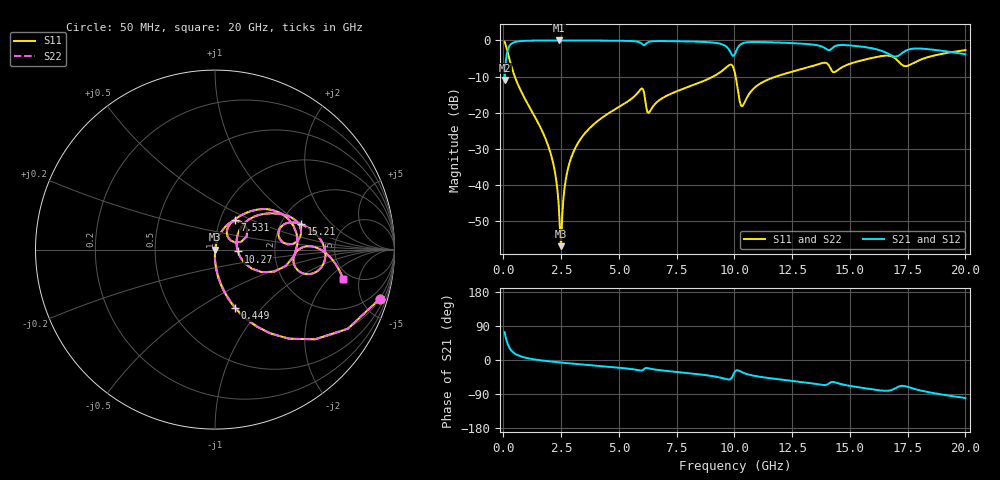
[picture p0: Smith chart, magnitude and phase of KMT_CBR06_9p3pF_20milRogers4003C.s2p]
! Data measured by Modelithics Inc. support@modelithics.com 813-866-6335
! KEMET CBR0603 9.3pF, Pad Width= 0.851mm, Pad Length= 0.64mm, Pad Gap= 0.62mm, 20mil Rogers 4003C substrate Data, January 2022
# hz S ma R 50
! 2 Port Network Data from SP1.SP block
! freq  magS11  angS11  magS21  angS21  magS12  angS12  magS22  angS22
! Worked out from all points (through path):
!   401 points, 50 MHz to 20 GHz, reference 50 ohm
!   highest |S21| = -0.01 dB at 2.394 GHz (marker M1); lowest = -11.0 dB at 50 MHz (marker M2)
!   group delay of S21, straight-line fit = 14.5 ps
!   lowest |S11| = -57.0 dB at 2.494 GHz (marker M3), VSWR 1.00, Z = 50.1 + j0.0514 ohm
!   |S11| at or under -10 dB: 489.8 MHz to 9.08 GHz (8.59 GHz wide, 180 % of centre); 10.05 GHz to 11.81 GHz (1.753 GHz wide, 16 % of centre)
!   |S22| runs from -57.0 to -0.4 dB; largest |S21 - S12| = 0
!   S11 on the Smith chart (normalised r, x): 50 MHz: 0.99, -6.73; 449 MHz: 0.99, -0.73; 7.531 GHz: 1.17, +0.41; 10.27 GHz: 1.29, -0.03; 15.21 GHz: 2.57, +0.97; 20 GHz: 4.24, -3.05
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5e7  0.9591 -16.6  0.2826 73.4  0.2826 73.4  0.9591 -16.6
2.495e8  0.5584 -56.7  0.8288 33.3  0.8288 33.3  0.5584 -56.7
4.49e8  0.3435 -71.0  0.9384 18.9  0.9384 18.9  0.3435 -71.0
1.94525e9  0.03417 -91.4  0.9982 -3.3  0.9982 -3.3  0.03417 -91.4
2.2445e9  0.01412 -90.4  0.9986 -5.3  0.9986 -5.3  0.01412 -90.4
2.394125e9  0.005202 -82.5  0.9987 -6.2  0.9987 -6.2  0.005202 -82.5
2.493875e9  0.001418 21.2  0.9987 -6.8  0.9987 -6.8  0.001418 21.2
2.843e9  0.01932 77.3  0.9984 -8.8  0.9984 -8.8  0.01932 77.3
3.391625e9  0.04567 76.4  0.9974 -11.8  0.9974 -11.8  0.04567 76.4
5.93525e9  0.2096 48.0  0.9271 -27.7  0.9271 -27.7  0.2096 48.0
6.284375e9  0.09914 40.8  0.9506 -22.0  0.9506 -22.0  0.09914 40.8
6.73325e9  0.1477 59.8  0.9796 -26.6  0.9796 -26.6  0.1477 59.8
7.53125e9  0.1993 56.8  0.9745 -31.7  0.9745 -31.7  0.1993 56.8
9.52625e9  0.3924 33.8  0.8682 -48.5  0.8682 -48.5  0.3924 33.8
1.0025e10  0.3518 -20.4  0.6513 -30.4  0.6513 -30.4  0.3518 -20.4
1.027438e10  0.1275 -4.8  0.8834 -30.7  0.8834 -30.7  0.1275 -4.8
1.336662e10  0.4412 25.5  0.877 -61.9  0.877 -61.9  0.4412 25.5
1.416462e10  0.4075 4.1  0.7473 -59.1  0.7473 -59.1  0.4075 4.1
1.5212e10  0.4987 16.5  0.84 -70.4  0.84 -70.4  0.4987 16.5
1.670825e10  0.6124 -6.4  0.6404 -80.6  0.6404 -80.6  0.6124 -6.4
1.74065e10  0.4403 -6.7  0.7173 -69.3  0.7173 -69.3  0.4403 -6.7
2e10  0.7337 -13.1  0.6437 -100.3  0.6437 -100.3  0.7337 -13.1
